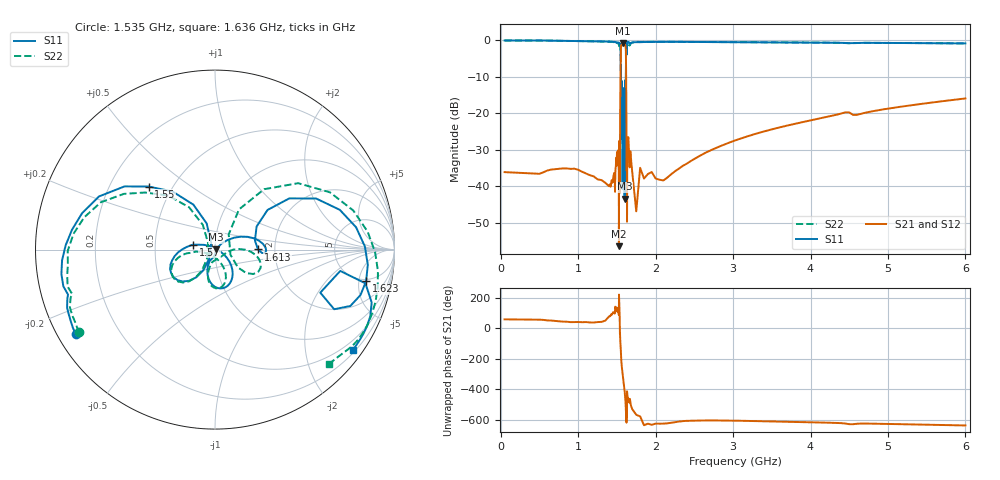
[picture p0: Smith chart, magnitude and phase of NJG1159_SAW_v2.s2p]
! Created Mon Mar 05 13:45:15 2018
# hz S ma R 50
! 2 Port Network Data from SP6.SP block
! freq  magS11  angS11  magS21  angS21  magS12  angS12  magS22  angS22
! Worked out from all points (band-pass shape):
!   414 points, 50 MHz to 6 GHz, reference 50 ohm
!   highest |S21| = -0.78 dB at 1.576 GHz (marker M1); lowest = -56.3 dB at 1.526 GHz (marker M2)
!   |S21| within 3 dB of the highest: 1.551 GHz to 1.616 GHz (65.98 MHz wide, 4.17 % of centre)
!   lowest |S11| = -43.4 dB at 1.6 GHz (marker M3), VSWR 1.01, Z = 50.7 + j0.139 ohm
!   |S11| at or under -10 dB: 1.552 GHz to 1.616 GHz (63.9 MHz wide, 4.04 % of centre)
!   |S22| runs from -28.1 to -0.1 dB; largest |S21 - S12| = 2.1e-09
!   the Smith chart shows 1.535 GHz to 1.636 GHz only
!   S11 on the Smith chart (normalised r, x): 1.535 GHz: 0.05, -0.28; 1.55 GHz: 0.37, +0.35; 1.57 GHz: 0.78, +0.04; 1.613 GHz: 1.63, +0.00; 1.623 GHz: 4.66, -6.29; 1.636 GHz: 0.27, -3.05
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5e7  0.9876 -34.3  0.01568 57.6  0.01568 57.6  0.9873 -36.3
1.5e8  0.9876 -34.8  0.01551 57.1  0.01551 57.1  0.9874 -36.9
2.5e8  0.9876 -35.4  0.01533 56.6  0.01533 56.6  0.9874 -37.5
5.5e8  0.9858 -40.1  0.0156 54.0  0.0156 54.0  0.986 -42.4
1.25e9  0.9592 -83.6  0.01248 39.7  0.01248 39.7  0.9579 -87.3
1.519e9  0.9254 -129.4  0.03132 122.3  0.03132 122.3  0.904 -130.8
1.526e9  0.9157 -136.9  0.001526 116.4  0.001526 116.4  0.8861 -140.3
1.53e9  0.8945 -140.3  0.04191 168.0  0.04191 168.0  0.8289 -140.5
1.535e9  0.9071 -148.8  0.01694 104.2  0.01694 104.2  0.8865 -148.7
1.55e9  0.51 136.5  0.6042 -137.9  0.6042 -137.9  0.5027 140.7
1.555e9  0.06013 -123.0  0.8445 162.2  0.8445 162.2  0.06872 -130.8
1.57e9  0.1257 167.4  0.8921 76.8  0.8921 76.8  0.1353 -172.4
1.576e9  0.0531 -27.6  0.9146 49.6  0.9146 49.6  0.0607 -73.4
1.588e9  0.2184 -82.2  0.898 0.5  0.898 0.5  0.2154 -88.9
1.6e9  0.006782 11.7  0.8982 -52.3  0.8982 -52.3  0.05525 -35.1
1.613e9  0.2395 0.3  0.8067 -140.0  0.8067 -140.0  0.162 -37.9
1.623e9  0.8601 -11.8  0.09547 103.4  0.09547 103.4  0.9154 -7.4
1.63e9  0.9212 -18.6  0.006561 136.3  0.006561 136.3  0.9341 -35.2
1.636e9  0.9493 -36.1  0.03535 -81.9  0.03535 -81.9  0.9003 -45.0
1.85e9  0.9404 -91.6  0.01282 83.8  0.01282 83.8  0.944 -95.4
2.75e9  0.9383 -124.9  0.03249 115.4  0.03249 115.4  0.9387 -128.1
6e9  0.8999 -176.1  0.1593 82.4  0.1593 82.4  0.9003 -177.3
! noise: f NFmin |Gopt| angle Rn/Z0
5e+07  6.369  0.9802  34.33  94.13
1.418e+09  20.34  0.9526  98.97  470.6
1.464e+09  17.26  0.9468  106.9  173.2
1.51e+09  17.46  0.9226  122.6  80.11
1.556e+09  1.385  0.07608  142.8  0.1449
1.602e+09  0.8851  0.07268  33.41  0.1165
1.648e+09  11.33  0.9212  51.02  67.23
1.694e+09  18.84  0.9243  70.72  324.1
3.7e+09  7.513  0.9076  143.8  2.793
6e+09  4.175  0.8328  172.8  0.07516
